| / 7\'7   Xilinx CoolRunner XPLA3 I/O Buffer IBIS File
| \ \   Xilinx Inc.
| / /   2100 Logic Drive
| \_\/.\   San Jose,   CA 95124
[IBIS ver]   2.1
[File name]   xcr3kxl.ibs
[File Rev]   0.6
[Date]   Aug 5, 2002
[Source]   Spice netlist
[Notes]   - Control flag setting:
   SLW=0 - fast slew rate
   SEW=1 - slow slew rate
[Disclaimer] The data in this model is derived from SPICE simulations using
   modeling information extracted from the target process. While
   a great deal of care has been take to provide information that
   is accurate, this model is considered preliminary as it has
   not been verified by actual silicon measurement. Treat the
   data in this model as preliminary until actual silicon
   verification is performed.
[Copyright]   Xilinx Inc. All right reserved
|   Component XCR3032XL_PC44[SLW=0]
[Component]   XCR3032XL_PC44[SLW=0]
[Manufacturer]   Xilinx Inc.
[Package]
| variable   typ   min   max
R_pkg   67.500m   66.000m   69.000m
L_pkg   3.950nH   3.600nH   4.300nH
C_pkg   0.900pF   0.800pF   1.000pF
[Pin]  signal_name   model_name   R_pin   L_pin   C_pin
io   PIN   IO_00   NA   NA   NA
| End [Component] XCR3032XL_PC44[SLW=0]
|   Component XCR3032XL_PC44[SLW=1]
[Component]   XCR3032XL_PC44[SLW=1]
[Manufacturer]   Xilinx Inc.
[Package]
| variable   typ   min   max
R_pkg   67.500m   66.000m   69.000m
L_pkg   3.950nH   3.600nH   4.300nH
C_pkg   0.900pF   0.800pF   1.000pF
[Pin]  signal_name   model_name   R_pin   L_pin   C_pin
io   PIN   IO_01   NA   NA   NA
| End [Component] XCR3032XL_PC44[SLW=1]
|   Component XCR3032XL_VQ44[SLW=0]
[Component]   XCR3032XL_VQ44[SLW=0]
[Manufacturer]   Xilinx Inc.
[Package]
| variable   typ   min   max
R_pkg   57.000m   54.000m   60.000m
L_pkg   2.250nH   2.100nH   2.400nH
C_pkg   0.300pF   0.300pF   0.300pF
[Pin]  signal_name   model_name   R_pin   L_pin   C_pin
io   PIN   IO_00   NA   NA   NA
| End [Component] XCR3032XL_VQ44[SLW=0]
|   Component XCR3032XL_VQ44[SLW=1]
[Component]   XCR3032XL_VQ44[SLW=1]
[Manufacturer]   Xilinx Inc.
[Package]
| variable   typ   min   max
R_pkg   57.000m   54.000m   60.000m
L_pkg   2.250nH   2.100nH   2.400nH
C_pkg   0.300pF   0.300pF   0.300pF
[Pin]  signal_name   model_name   R_pin   L_pin   C_pin
io   PIN   IO_01   NA   NA   NA
| End [Component] XCR3032XL_VQ44[SLW=1]
|   Component XCR3032XL_CS48[SLW=0]
[Component]   XCR3032XL_CS48[SLW=0]
[Manufacturer]   Xilinx Inc.
[Package]
| variable   typ   min   max
R_pkg   62.000m   26.000m   98.000m
L_pkg   2.100nH   1.800nH   2.400nH
C_pkg   0.250pF   0.200pF   0.300pF
[Pin]  signal_name   model_name   R_pin   L_pin   C_pin
io   PIN   IO_00   NA   NA   NA
| End [Component] XCR3032XL_CS48[SLW=0]
|   Component XCR3032XL_CS48[SLW=1]
[Component]   XCR3032XL_CS48[SLW=1]
[Manufacturer]   Xilinx Inc.
[Package]
| variable   typ   min   max
R_pkg   62.000m   26.000m   98.000m
L_pkg   2.100nH   1.800nH   2.400nH
C_pkg   0.250pF   0.200pF   0.300pF
[Pin]  signal_name   model_name   R_pin   L_pin   C_pin
io   PIN   IO_01   NA   NA   NA
| End [Component] XCR3032XL_CS48[SLW=1]
|   Component XCR3064XL_PC44[SLW=0]
[Component]   XCR3064XL_PC44[SLW=0]
[Manufacturer]   Xilinx Inc.
[Package]
| variable   typ   min   max
R_pkg   64.500m   63.000m   66.000m
L_pkg   3.750nH   3.400nH   4.100nH
C_pkg   0.900pF   0.800pF   1.000pF
[Pin]  signal_name   model_name   R_pin   L_pin   C_pin
io   PIN   IO_00   NA   NA   NA
| End [Component] XCR3064XL_PC44[SLW=0]
|   Component XCR3064XL_PC44[SLW=1]
[Component]   XCR3064XL_PC44[SLW=1]
[Manufacturer]   Xilinx Inc.
[Package]
| variable   typ   min   max
R_pkg   64.500m   63.000m   66.000m
L_pkg   3.750nH   3.400nH   4.100nH
C_pkg   0.900pF   0.800pF   1.000pF
[Pin]  signal_name   model_name   R_pin   L_pin   C_pin
io   PIN   IO_01   NA   NA   NA
| End [Component] XCR3064XL_PC44[SLW=1]
|   Component XCR3064XL_CP56[SLW=0]
[Component]   XCR3064XL_CP56[SLW=0]
[Manufacturer]   Xilinx Inc.
[Package]
| variable   typ   min   max
R_pkg   89.000m   75.000m   103.000m
L_pkg   1.850nH   1.500nH   2.200nH
C_pkg   0.350pF   0.300pF   0.400pF
[Pin]  signal_name   model_name   R_pin   L_pin   C_pin
io   PIN   IO_00   NA   NA   NA
| End [Component] XCR3064XL_CP56[SLW=0]
|   Component XCR3064XL_CP56[SLW=1]
[Component]   XCR3064XL_CP56[SLW=1]
[Manufacturer]   Xilinx Inc.
[Package]
| variable   typ   min   max
R_pkg   89.000m   75.000m   103.000m
L_pkg   1.850nH   1.500nH   2.200nH
C_pkg   0.350pF   0.300pF   0.400pF
[Pin]  signal_name   model_name   R_pin   L_pin   C_pin
io   PIN   IO_01   NA   NA   NA
| End [Component] XCR3064XL_CP56[SLW=1]
|   Component XCR3064XL_CS48[SLW=0]
[Component]   XCR3064XL_CS48[SLW=0]
[Manufacturer]   Xilinx Inc.
[Package]
| variable   typ   min   max
R_pkg   112.000m   98.000m   126.000m
L_pkg   2.100nH   1.800nH   2.400nH
C_pkg   0.250pF   0.200pF   0.300pF
[Pin]  signal_name   model_name   R_pin   L_pin   C_pin
io   PIN   IO_00   NA   NA   NA
| End [Component] XCR3064XL_CS48[SLW=0]
|   Component XCR3064XL_CS48[SLW=1]
[Component]   XCR3064XL_CS48[SLW=1]
[Manufacturer]   Xilinx Inc.
[Package]
| variable   typ   min   max
R_pkg   112.000m   98.000m   126.000m
L_pkg   2.100nH   1.800nH   2.400nH
C_pkg   0.250pF   0.200pF   0.300pF
[Pin]  signal_name   model_name   R_pin   L_pin   C_pin
io   PIN   IO_01   NA   NA   NA
| End [Component] XCR3064XL_CS48[SLW=1]
|   Component XCR3064XL_VQ44[SLW=0]
[Component]   XCR3064XL_VQ44[SLW=0]
[Manufacturer]   Xilinx Inc.
[Package]
| variable   typ   min   max
R_pkg   57.000m   54.000m   60.000m
L_pkg   2.250nH   2.100nH   2.400nH
C_pkg   0.300pF   0.300pF   0.300pF
[Pin]  signal_name   model_name   R_pin   L_pin   C_pin
io   PIN   IO_00   NA   NA   NA
| End [Component] XCR3064XL_VQ44[SLW=0]
|   Component XCR3064XL_VQ44[SLW=1]
[Component]   XCR3064XL_VQ44[SLW=1]
[Manufacturer]   Xilinx Inc.
[Package]
| variable   typ   min   max
R_pkg   57.000m   54.000m   60.000m
L_pkg   2.250nH   2.100nH   2.400nH
C_pkg   0.300pF   0.300pF   0.300pF
[Pin]  signal_name   model_name   R_pin   L_pin   C_pin
io   PIN   IO_01   NA   NA   NA
| End [Component] XCR3064XL_VQ44[SLW=1]
|   Component XCR3064XL_VQ100[SLW=0]
[Component]   XCR3064XL_VQ100[SLW=0]
[Manufacturer]   Xilinx Inc.
[Package]
| variable   typ   min   max
R_pkg   101.500m   98.000m   105.000m
L_pkg   5.200nH   4.700nH   5.700nH
C_pkg   0.550pF   0.400pF   0.700pF
[Pin]  signal_name   model_name   R_pin   L_pin   C_pin
io   PIN   IO_00   NA   NA   NA
| End [Component] XCR3064XL_VQ100[SLW=0]
|   Component XCR3064XL_VQ100[SLW=1]
[Component]   XCR3064XL_VQ100[SLW=1]
[Manufacturer]   Xilinx Inc.
[Package]
| variable   typ   min   max
R_pkg   101.500m   98.000m   105.000m
L_pkg   5.200nH   4.700nH   5.700nH
C_pkg   0.550pF   0.400pF   0.700pF
[Pin]  signal_name   model_name   R_pin   L_pin   C_pin
io   PIN   IO_01   NA   NA   NA
| End [Component] XCR3064XL_VQ100[SLW=1]
|   Component XCR3128XL_CS144[SLW=0]
[Component]   XCR3128XL_CS144[SLW=0]
[Manufacturer]   Xilinx Inc.
[Package]
| variable   typ   min   max
R_pkg   109.500m   76.000m   143.000m
L_pkg   2.250nH   1.500nH   3.000nH
C_pkg   0.250pF   0.200pF   0.300pF
[Pin]  signal_name   model_name   R_pin   L_pin   C_pin
io   PIN   IO_00   NA   NA   NA
| End [Component] XCR3128XL_CS144[SLW=0]
|   Component XCR3128XL_CS144[SLW=1]
[Component]   XCR3128XL_CS144[SLW=1]
[Manufacturer]   Xilinx Inc.
[Package]
| variable   typ   min   max
R_pkg   109.500m   76.000m   143.000m
L_pkg   2.250nH   1.500nH   3.000nH
C_pkg   0.250pF   0.200pF   0.300pF
[Pin]  signal_name   model_name   R_pin   L_pin   C_pin
io   PIN   IO_01   NA   NA   NA
| End [Component] XCR3128XL_CS144[SLW=1]
|   Component XCR3128XL_TQ144[SLW=0]
[Component]   XCR3128XL_TQ144[SLW=0]
[Manufacturer]   Xilinx Inc.
[Package]
| variable   typ   min   max
R_pkg   123.500m   117.000m   130.000m
L_pkg   7.950nH   7.100nH   8.800nH
C_pkg   1.000pF   0.800pF   1.200pF
[Pin]  signal_name   model_name   R_pin   L_pin   C_pin
io   PIN   IO_00   NA   NA   NA
| End [Component] XCR3128XL_TQ144[SLW=0]
|   Component XCR3128XL_TQ144[SLW=1]
[Component]   XCR3128XL_TQ144[SLW=1]
[Manufacturer]   Xilinx Inc.
[Package]
| variable   typ   min   max
R_pkg   123.500m   117.000m   130.000m
L_pkg   7.950nH   7.100nH   8.800nH
C_pkg   1.000pF   0.800pF   1.200pF
[Pin]  signal_name   model_name   R_pin   L_pin   C_pin
io   PIN   IO_01   NA   NA   NA
| End [Component] XCR3128XL_TQ144[SLW=1]
|   Component XCR3128XL_VQ100[SLW=0]
[Component]   XCR3128XL_VQ100[SLW=0]
[Manufacturer]   Xilinx Inc.
[Package]
| variable   typ   min   max
R_pkg   101.500m   98.000m   105.000m
L_pkg   5.200nH   4.700nH   5.700nH
C_pkg   0.550pF   0.400pF   0.700pF
[Pin]  signal_name   model_name   R_pin   L_pin   C_pin
io   PIN   IO_00   NA   NA   NA
| End [Component] XCR3128XL_VQ100[SLW=0]
|   Component XCR3128XL_VQ100[SLW=1]
[Component]   XCR3128XL_VQ100[SLW=1]
[Manufacturer]   Xilinx Inc.
[Package]
| variable   typ   min   max
R_pkg   101.500m   98.000m   105.000m
L_pkg   5.200nH   4.700nH   5.700nH
C_pkg   0.550pF   0.400pF   0.700pF
[Pin]  signal_name   model_name   R_pin   L_pin   C_pin
io   PIN   IO_01   NA   NA   NA
| End [Component] XCR3128XL_VQ100[SLW=1]
|   Component XCR3256XL_CS280[SLW=0]
[Component]   XCR3256XL_CS280[SLW=0]
[Manufacturer]   Xilinx Inc.
[Package]
| variable   typ   min   max
R_pkg   259.500m   148.000m   371.000m
L_pkg   5.800nH   2.700nH   8.900nH
C_pkg   0.500pF   0.200pF   0.800pF
[Pin]  signal_name   model_name   R_pin   L_pin   C_pin
io   PIN   IO_00   NA   NA   NA
| End [Component] XCR3256XL_CS280[SLW=0]
|   Component XCR3256XL_CS280[SLW=1]
[Component]   XCR3256XL_CS280[SLW=1]
[Manufacturer]   Xilinx Inc.
[Package]
| variable   typ   min   max
R_pkg   259.500m   148.000m   371.000m
L_pkg   5.800nH   2.700nH   8.900nH
C_pkg   0.500pF   0.200pF   0.800pF
[Pin]  signal_name   model_name   R_pin   L_pin   C_pin
io   PIN   IO_01   NA   NA   NA
| End [Component] XCR3256XL_CS280[SLW=1]
|   Component XCR3256XL_PQ208[SLW=0]
[Component]   XCR3256XL_PQ208[SLW=0]
[Manufacturer]   Xilinx Inc.
[Package]
| variable   typ   min   max
R_pkg   195.500m   195.000m   196.000m
L_pkg   14.200nH   12.500nH   15.900nH
C_pkg   1.800pF   1.600pF   2.000pF
[Pin]  signal_name   model_name   R_pin   L_pin   C_pin
io   PIN   IO_00   NA   NA   NA
| End [Component] XCR3256XL_PQ208[SLW=0]
|   Component XCR3256XL_PQ208[SLW=1]
[Component]   XCR3256XL_PQ208[SLW=1]
[Manufacturer]   Xilinx Inc.
[Package]
| variable   typ   min   max
R_pkg   195.500m   195.000m   196.000m
L_pkg   14.200nH   12.500nH   15.900nH
C_pkg   1.800pF   1.600pF   2.000pF
[Pin]  signal_name   model_name   R_pin   L_pin   C_pin
io   PIN   IO_01   NA   NA   NA
| End [Component] XCR3256XL_PQ208[SLW=1]
|   Component XCR3256XL_TQ144[SLW=0]
[Component]   XCR3256XL_TQ144[SLW=0]
[Manufacturer]   Xilinx Inc.
[Package]
| variable   typ   min   max
R_pkg   123.500m   117.000m   130.000m
L_pkg   7.950nH   7.100nH   8.800nH
C_pkg   1.000pF   0.800pF   1.200pF
[Pin]  signal_name   model_name   R_pin   L_pin   C_pin
io   PIN   IO_00   NA   NA   NA
| End [Component] XCR3256XL_TQ144[SLW=0]
|   Component XCR3256XL_TQ144[SLW=1]
[Component]   XCR3256XL_TQ144[SLW=1]
[Manufacturer]   Xilinx Inc.
[Package]
| variable   typ   min   max
R_pkg   123.500m   117.000m   130.000m
L_pkg   7.950nH   7.100nH   8.800nH
C_pkg   1.000pF   0.800pF   1.200pF
[Pin]  signal_name   model_name   R_pin   L_pin   C_pin
io   PIN   IO_01   NA   NA   NA
| End [Component] XCR3256XL_TQ144[SLW=1]
|   Component XCR3256XL_FT256[SLW=0]
[Component]   XCR3256XL_FT256[SLW=0]
[Manufacturer]   Xilinx Inc.
[Package]
| variable   typ   min   max
R_pkg   229.500m   194.000m   265.000m
L_pkg   4.950nH   3.000nH   6.900nH
C_pkg   0.900pF   0.600pF   1.200pF
[Pin]  signal_name   model_name   R_pin   L_pin   C_pin
io   PIN   IO_00   NA   NA   NA
| End [Component] XCR3256XL_TQ144[SLW=0]
|   Component XCR3256XL_FT256[SLW=1]
[Component]   XCR3256XL_FT256[SLW=1]
[Manufacturer]   Xilinx Inc.
[Package]
| variable   typ   min   max
R_pkg   229.500m   194.000m   265.000m
L_pkg   4.950nH   3.000nH   6.900nH
C_pkg   0.900pF   0.600pF   1.200pF
[Pin]  signal_name   model_name   R_pin   L_pin   C_pin
io   PIN   IO_01   NA   NA   NA
| End [Component] XCR3256XL_FT256[SLW=1]
|   Component XCR3384XL_PQ208[SLW=0]
[Component]   XCR3384XL_PQ208[SLW=0]
[Manufacturer]   Xilinx Inc.
[Package]
| variable   typ   min   max
R_pkg   187.500m   180.000m   195.000m
L_pkg   12.100nH   11.700nH   12.500nH
C_pkg   1.4500pF   1.3000pF   1.6000pF
[Pin]  signal_name   model_name   R_pin   L_pin   C_pin
io   PIN   IO_00   NA   NA   NA
| End [Component] XCR3384XL_PQ208[SLW=0]
|   Component XCR3384XL_PQ208[SLW=1]
[Component]   XCR3384XL_PQ208[SLW=1]
[Manufacturer]   Xilinx Inc.
[Package]
| variable   typ   min   max
R_pkg   187.500m   180.000m   195.000m
L_pkg   12.100nH   11.700nH   12.500nH
C_pkg   1.4500pF   1.3000pF   1.6000pF
[Pin]  signal_name   model_name   R_pin   L_pin   C_pin
io   PIN   IO_01   NA   NA   NA
| End [Component] XCR3384XL_PQ208[SLW=1]
|   Component XCR3384XL_FT256[SLW=0]
[Component]   XCR3384XL_FT256[SLW=0]
[Manufacturer]   Xilinx Inc.
[Package]
| variable   typ   min   max
R_pkg   266.950m   201.300m   332.600m
L_pkg   6.5500nH   3.2000nH   9.9000nH
C_pkg   0.9500pF   0.6000pF   1.3000pF
[Pin]  signal_name   model_name   R_pin   L_pin   C_pin
io   PIN   IO_00   NA   NA   NA
| End [Component] XCR3384XL_FT256[SLW=0]
|   Component XCR3384XL_FT256[SLW=1]
[Component]   XCR3384XL_FT256[SLW=1]
[Manufacturer]   Xilinx Inc.
[Package]
| variable   typ   min   max
R_pkg   266.950m   201.300m   332.600m
L_pkg   6.5500nH   3.2000nH   9.9000nH
C_pkg   0.9500pF   0.6000pF   1.3000pF
[Pin]  signal_name   model_name   R_pin   L_pin   C_pin
io   PIN   IO_01   NA   NA   NA
| End [Component] XCR3384XL_FT256[SLW=1]
|   Component XCR3384XL_FG324[SLW=0]
[Component]   XCR3384XL_FG324[SLW=0]
[Manufacturer]   Xilinx Inc.
[Package]
| variable   typ   min   max
R_pkg   293.000m   233.000m   353.000m
L_pkg   6.0500nH   3.9000nH   8.2000nH
C_pkg   1.6000pF   1.3000pF   1.9000pF
[Pin]  signal_name   model_name   R_pin   L_pin   C_pin
io   PIN   IO_00   NA   NA   NA
| End [Component] XCR3384XL_FG324[SLW=0]
|   Component XCR3384XL_FG324[SLW=1]
[Component]   XCR3384XL_FG324[SLW=1]
[Manufacturer]   Xilinx Inc.
[Package]
| variable   typ   min   max
R_pkg   293.000m   233.000m   353.000m
L_pkg   6.0500nH   3.9000nH   8.2000nH
C_pkg   1.6000pF   1.3000pF   1.9000pF
[Pin]  signal_name   model_name   R_pin   L_pin   C_pin
io   PIN   IO_01   NA   NA   NA
| End [Component] XCR3384XL_FG324[SLW=1]
|   Component XCR3384XL_TQ144[SLW=0]
[Component]   XCR3384XL_TQ144[SLW=0]
[Manufacturer]   Xilinx Inc.
[Package]
| variable   typ   min   max
R_pkg   123.500m   117.000m   130.000m
L_pkg   7.9500nH   7.1000nH   8.8000nH
C_pkg   1.0000pF   0.8000pF   1.2000pF
[Pin]  signal_name   model_name   R_pin   L_pin   C_pin
io   PIN   IO_00   NA   NA   NA
| End [Component] XCR3384XL_TQ144[SLW=0]
|   Component XCR3384XL_TQ144[SLW=1]
[Component]   XCR3384XL_TQ144[SLW=1]
[Manufacturer]   Xilinx Inc.
[Package]
| variable   typ   min   max
R_pkg   123.500m   117.000m   130.000m
L_pkg   7.9500nH   7.1000nH   8.8000nH
C_pkg   1.0000pF   0.8000pF   1.2000pF
[Pin]  signal_name   model_name   R_pin   L_pin   C_pin
io   PIN   IO_01   NA   NA   NA
| End [Component] XCR3384XL_TQ144[SLW=1]
|   Component XCR3512XL_PQ208[SLW=0]
[Component]   XCR3512XL_PQ208[SLW=0]
[Manufacturer]   Xilinx Inc.
[Package]
| variable   typ   min   max
R_pkg   178.500m   176.000m   181.000m
L_pkg   13.100nH   11.500nH   14.700nH
C_pkg   1.5500pF   1.3000pF   1.8000pF
[Pin]  signal_name   model_name   R_pin   L_pin   C_pin
io   PIN   IO_00   NA   NA   NA
| End [Component] XCR3512XL_PQ208[SLW=0]
|   Component XCR3512XL_PQ208[SLW=1]
[Component]   XCR3512XL_PQ208[SLW=1]
[Manufacturer]   Xilinx Inc.
[Package]
| variable   typ   min   max
R_pkg   178.500m   176.000m   181.000m
L_pkg   13.100nH   11.500nH   14.700nH
C_pkg   1.5500pF   1.3000pF   1.8000pF
[Pin]  signal_name   model_name   R_pin   L_pin   C_pin
io   PIN   IO_01   NA   NA   NA
| End [Component] XCR3512XL_PQ208[SLW=1]
|   Component XCR3512XL_FT256[SLW=0]
[Component]   XCR3512XL_FT256[SLW=0]
[Manufacturer]   Xilinx Inc.
[Package]
| variable   typ   min   max
R_pkg   207.000m   175.000m   239.000m
L_pkg   4.4500nH   2.7000nH   6.2000nH
C_pkg   0.8000pF   0.5000pF   1.1000pF
[Pin]  signal_name   model_name   R_pin   L_pin   C_pin
io   PIN   IO_00   NA   NA   NA
| End [Component] XCR3512XL_FT256[SLW=0]
|   Component XCR3512XL_FT256[SLW=1]
[Component]   XCR3512XL_FT256[SLW=1]
[Manufacturer]   Xilinx Inc.
[Package]
| variable   typ   min   max
R_pkg   207.000m   175.000m   239.000m
L_pkg   4.4500nH   2.7000nH   6.2000nH
C_pkg   0.8000pF   0.5000pF   1.1000pF
[Pin]  signal_name   model_name   R_pin   L_pin   C_pin
io   PIN   IO_01   NA   NA   NA
| End [Component] XCR3512XL_FT256[SLW=1]
| Models and submodels in the file (2): IO_00 (I/O), IO_01 (I/O)
